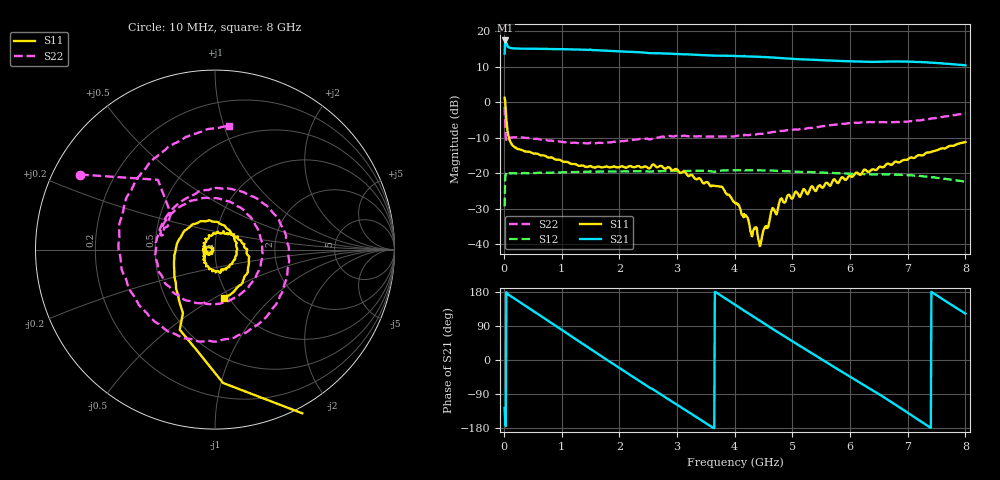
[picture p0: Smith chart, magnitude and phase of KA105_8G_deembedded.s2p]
!Agilent	"Technologies,N5230A,MY45001650,A.07.50.48"
!Agilent	N5230A:	A.07.50.48
!Date:	"Monday,"	April	"09,"	2018	11:21:49
!Correction:	S11(Full	2	"Port(1,2))"
!S21(Full	2	"Port(1,2))"
!S12(Full	2	"Port(1,2))"
!S22(Full	2	"Port(1,2))"
!S2P	File:	Measurements:	"S11,"	"S21,"	"S12,"	S22:
#	Hz	S	dB	R	50
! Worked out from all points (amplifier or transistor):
!   801 points, 10 MHz to 8 GHz, reference 50 ohm
!   highest |S21| = 17.4 dB at 19.99 MHz (marker M1)
!   |S21| within 3 dB of that: 11.86 MHz to 1.946 GHz (1.934 GHz wide, 198 % of centre)
!   unconditionally stable (mu >= 1): 54.82 MHz to end of sweep
!   at 1.338 GHz: K = 1.11, MAG = 15.2 dB, |S12| = -19.7 dB
!   at 4.005 GHz: K = 1.15, MAG = 13.7 dB, |S12| = -19.2 dB
!   at 8 GHz: K = 1.28, MAG = 13.2 dB, |S12| = -22.5 dB
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1e7  1.22 -23.0  13.67 -126.7  -29.35 119.4  -1.31 150.9
1.99875e7  0.29 -61.9  17.35 -158.6  -21.67 71.3  -5.98 129.3
5.99375e7  -8.05 -116.8  15.71 175.3  -20.07 18.2  -10.51 163.2
8.99e7  -10.27 -135.0  15.36 171.2  -20.05 9.5  -10.19 165.3
6.29225e8  -14.99 124.5  14.99 117.1  -19.92 -45.0  -10.54 111.3
9.88775e8  -16.43 82.1  14.91 80.8  -19.78 -73.5  -11.14 68.8
1.348325e9  -17.84 36.5  14.76 44.3  -19.65 -102.4  -11.55 25.8
1.64795e9  -18.17 0.6  14.58 14.1  -19.57 -126.5  -11.46 -8.5
1.937588e9  -18.35 -28.3  14.36 -14.8  -19.50 -150.1  -11.22 -41.2
2.337088e9  -18.02 -60.7  14.04 -54.3  -19.47 177.7  -10.44 -83.0
2.676662e9  -18.24 -87.7  13.75 -86.7  -19.47 150.9  -9.99 -113.8
3.00625e9  -19.04 -106.8  13.51 -118.7  -19.39 124.0  -9.51 -148.1
3.3658e9  -21.45 -139.3  13.27 -153.6  -19.35 94.3  -9.63 174.4
3.705375e9  -23.70 -168.7  13.08 175.7  -19.42 68.3  -9.70 142.5
4.005e9  -28.43 155.0  12.98 145.7  -19.21 42.2  -9.64 109.1
4.624225e9  -31.49 -144.2  12.59 85.3  -19.28 -11.2  -8.56 42.8
5.343325e9  -23.71 179.6  11.93 17.2  -19.71 -72.1  -7.26 -27.0
5.672912e9  -23.17 133.9  11.70 -13.8  -19.91 -99.8  -6.49 -55.1
6.092388e9  -20.03 81.8  11.43 -52.7  -20.20 -135.3  -5.80 -89.6
6.671662e9  -17.34 39.3  11.40 -106.6  -20.37 174.9  -5.62 -142.0
7.330838e9  -14.23 -11.7  11.20 -172.2  -21.00 113.2  -4.87 146.2
8e9  -11.26 -80.0  10.35 122.5  -22.50 50.5  -3.18 83.6
